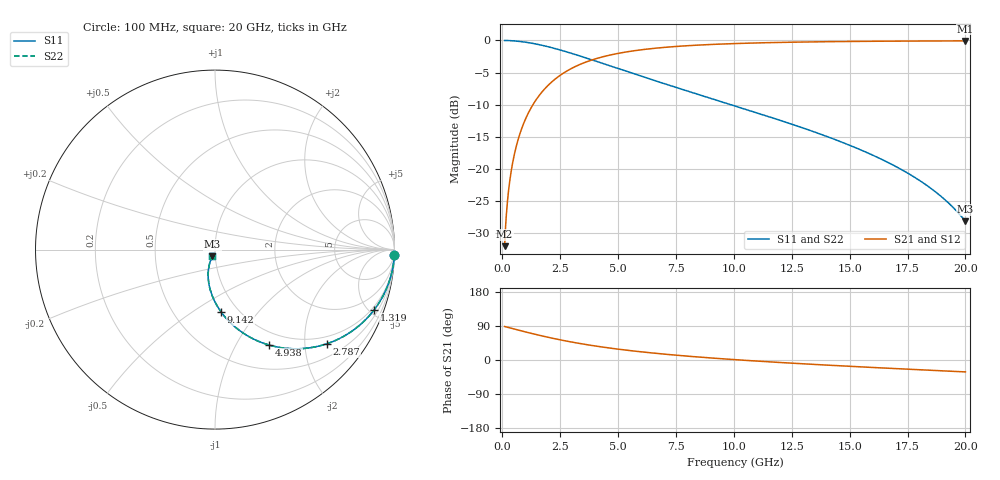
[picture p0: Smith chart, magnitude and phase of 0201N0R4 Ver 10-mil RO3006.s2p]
# GHz S MA R 50
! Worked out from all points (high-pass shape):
!   1601 points, 100 MHz to 20 GHz, reference 50 ohm
!   highest |S21| = -0.07 dB at 20 GHz (marker M1); lowest = -32.0 dB at 100 MHz (marker M2)
!   |S21| within 3 dB of the highest: 3.841 GHz to end of sweep
!   lowest |S11| = -28.1 dB at 20 GHz (marker M3), VSWR 1.08, Z = 48.5 - j3.55 ohm
!   |S11| at or under -10 dB: 9.892 GHz to end of sweep
!   |S22| runs from -28.1 to 0.0 dB; largest |S21 - S12| = 0
!   S11 on the Smith chart (normalised r, x): 100 MHz: 1, -71; 1.319 GHz: 0.80, -5.37; 2.787 GHz: 0.81, -2.51; 4.938 GHz: 0.81, -1.37; 9.142 GHz: 0.83, -0.66; 20 GHz: 0.97, -0.07
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0.1  0.9997 -1.6  0.02516 88.4  0.02516 88.4  0.9997 -1.6
0.1621875  0.9992 -2.6  0.04079 87.4  0.04079 87.4  0.9992 -2.6
0.24925  0.998 -4.0  0.06261 86.0  0.06261 86.0  0.998 -4.0
0.299  0.9972 -4.8  0.07505 85.2  0.07505 85.2  0.9972 -4.8
0.3985  0.995 -6.4  0.09981 83.6  0.09981 83.6  0.995 -6.4
0.522875  0.9914 -8.4  0.1305 81.6  0.1305 81.6  0.9914 -8.4
0.672125  0.9859 -10.8  0.1669 79.2  0.1669 79.2  0.9859 -10.8
0.8586875  0.9772 -13.7  0.2114 76.3  0.2114 76.3  0.9772 -13.7
1.318875  0.9485 -20.7  0.3157 69.3  0.3157 69.3  0.9485 -20.7
1.965625  0.8946 -29.8  0.4453 60.1  0.4453 60.1  0.8946 -29.8
2.7865  0.8144 -40.1  0.5783 49.7  0.5783 49.7  0.8144 -40.1
3.420812  0.7505 -47.1  0.6584 42.8  0.6584 42.8  0.7505 -47.1
4.938187  0.61 -60.6  0.7891 29.1  0.7891 29.1  0.61 -60.6
5.808813  0.5413 -66.8  0.8372 22.8  0.8372 22.8  0.5413 -66.8
6.741625  0.4772 -72.6  0.8747 17.0  0.8747 17.0  0.4772 -72.6
9.142062  0.3484 -84.5  0.9325 4.8  0.9325 4.8  0.3484 -84.5
10.05  0.3098 -88.2  0.9457 0.9  0.9457 0.9  0.3098 -88.2
13.37081  0.1975 -99.7  0.9744 -11.3  0.9744 -11.3  0.1975 -99.7
16.69162  0.1118 -108.6  0.9871 -21.8  0.9871 -21.8  0.1118 -108.6
18.56969  0.06954 -111.9  0.9905 -27.4  0.9905 -27.4  0.06954 -111.9
19.27863  0.05435 -112.2  0.9913 -29.4  0.9913 -29.4  0.05435 -112.2
20  0.03928 -111.3  0.9919 -31.4  0.9919 -31.4  0.03928 -111.3
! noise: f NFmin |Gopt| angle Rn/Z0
0.1  0.001293  0.9768  1.089  0.0127
2.301  0.005419  0.8316  5.67  0.006769
4.515  0.008315  0.787  9.169  0.00798
6.729  0.01082  0.7591  12.73  0.008988
8.943  0.01311  0.739  16.31  0.00986
11.14  0.01526  0.7235  19.85  0.01063
13.36  0.01732  0.7112  23.4  0.01135
15.57  0.01933  0.7012  26.91  0.01201
17.79  0.0213  0.6931  30.38  0.01263
20  0.02324  0.6866  33.81  0.01322
